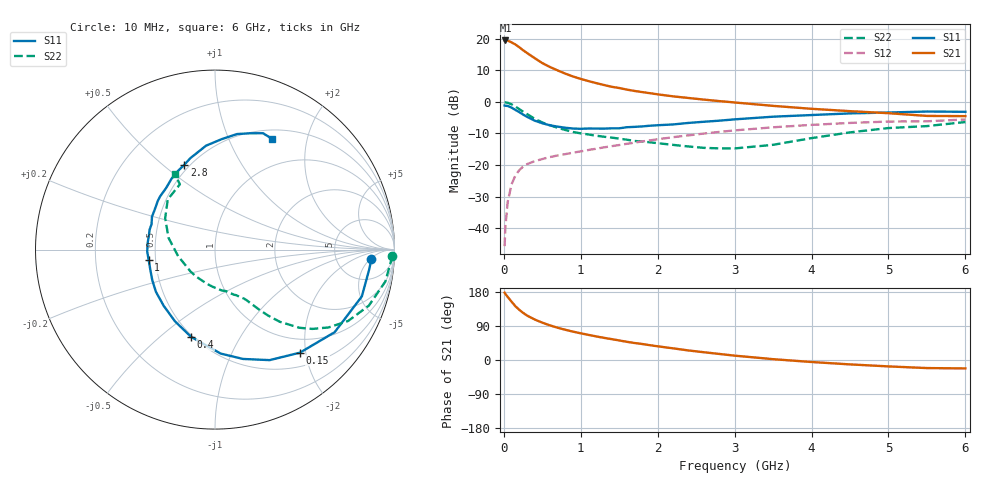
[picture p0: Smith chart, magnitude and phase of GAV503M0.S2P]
! Infineon Technologies  Discrete & RF Semiconductors
! BF775
! Si NPN RF Bipolar Junction Transistor in SOT23
! VCE = 0.5 V  IC = 3 mA
! Common Emitter S-Parameters:  May  1996
# GHz  S  MA  R  50
!  f  S11  S21  S12  S22
! GHz  MAG  ANG  MAG  ANG  MAG  ANG  MAG  ANG
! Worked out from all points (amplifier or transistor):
!   36 points, 10 MHz to 6 GHz, reference 50 ohm
!   highest |S21| = 19.4 dB at 20 MHz (marker M1)
!   |S21| within 3 dB of that: start of sweep to 245.5 MHz
!   unconditionally stable (mu >= 1): 830.3 MHz to end of sweep
!   at 250 MHz: K = 0.40, MSG = 18.4 dB, |S12| = -20.5 dB
!   at 1.4 GHz: K = 1.22, MAG = 6.6 dB, |S12| = -14.0 dB
!   at 6 GHz: K = 1.09, MAG = -1.3 dB, |S12| = -5.6 dB
!   S11 on the Smith chart (normalised r, x): 10 MHz: 12, -6; 150 MHz: 0.74, -1.89; 400 MHz: 0.49, -0.64; 1 GHz: 0.46, -0.06; 2.8 GHz: 0.47, +0.59; 6 GHz: 0.61, +1.46
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0.01  0.8725 -3.6  9.272 177.6  0.0052 85.3  0.9883 -2.0
0.02  0.8663 -7.3  9.341 174.4  0.0105 84.9  0.9812 -4.2
0.05  0.8587 -17.7  9.307 166.4  0.0259 80.2  0.9659 -10.6
0.1  0.8101 -34.6  8.705 154.1  0.0494 70.9  0.9122 -20.0
0.15  0.7441 -50.5  8.074 141.8  0.0681 62.5  0.8416 -28.2
0.2  0.6869 -63.7  7.311 132.6  0.0828 56.8  0.7674 -34.4
0.25  0.629 -75.6  6.548 124.5  0.0942 52.1  0.6992 -39.2
0.3  0.5801 -86.9  5.935 117.5  0.103 49.0  0.641 -42.8
0.4  0.5037 -105.4  4.913 107.0  0.115 44.7  0.5401 -48.1
0.5  0.4577 -119.1  4.096 98.5  0.1243 42.2  0.4706 -51.2
0.6  0.4242 -132.3  3.548 91.3  0.1337 41.2  0.425 -53.2
0.7  0.4046 -144.4  3.135 85.1  0.1416 40.6  0.3879 -54.9
0.8  0.3886 -154.1  2.785 79.7  0.1488 40.6  0.358 -56.5
1  0.3739 -170.9  2.3 70.4  0.1642 40.9  0.3167 -59.4
1.1  0.3779 -178.2  2.125 66.3  0.173 41.0  0.3039 -61.5
1.6  0.3961 152.4  1.558 48.0  0.2166 40.7  0.2513 -72.3
2.2  0.4382 128.4  1.219 30.7  0.2754 37.8  0.2083 -93.0
2.8  0.5027 109.9  1.026 16.0  0.3336 32.4  0.1834 -125.1
3.5  0.5813 94.9  0.862 2.2  0.3951 24.0  0.2087 -170.0
4.5  0.6554 79.2  0.711 -11.6  0.4631 11.4  0.3283 147.8
5.5  0.7014 67.6  0.598 -21.3  0.4916 -1.6  0.4126 118.3
6  0.6945 62.8  0.593 -22.2  0.5253 -5.1  0.4783 117.9
